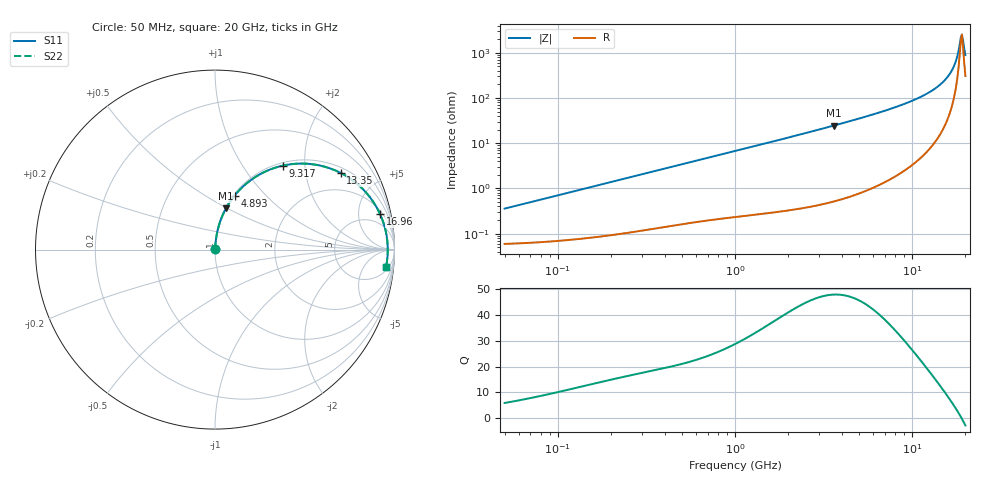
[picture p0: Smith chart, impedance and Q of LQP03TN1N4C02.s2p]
!Murata Part Number: LQP03TN1N4C02
!These Parameters are Measured in Series Mode Connection
!  o--[Z]--o
!Port1  Port2
!  o-------o
!Freq. Start=50[MHz] Stop=20[GHz], 401[Steps]
# Hz S RI R 50
!Freq.(Hz) S11(Real) S11(Imag) S21(Real) S21(Imag) S12(Real) S12(Imag) S22(Real) S22(Imag)
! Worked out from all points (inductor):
!   401 points, 50 MHz to 20 GHz, reference 50 ohm
!   read as one part in series: L = 1.12 nH near 51.52 MHz
!   highest Q = 47.7 at 3.626 GHz (marker M1), where L = 1.08 nH
!   self-resonance near 18.84 GHz
!   S11 on the Smith chart (normalised r, x): 50 MHz: 1.00, +0.01; 4.893 GHz: 1.01, +0.68; 9.317 GHz: 1.05, +1.55; 13.35 GHz: 1.20, +3.14; 16.96 GHz: 2.54, +8.71; 20 GHz: 7, -17
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5e7  0.000604 0.00352  0.9994 -0.00352  0.9994 -0.00352  0.000604 0.00352
1.364002e8  0.000862 0.00948  0.9991 -0.00948  0.9991 -0.00948  0.000862 0.00948
3.721004e8  0.00198 0.0253  0.998 -0.0253  0.998 -0.0253  0.00198 0.0253
1e9  0.00672 0.0661  0.9933 -0.0661  0.9933 -0.0661  0.00672 0.0661
2.728004e9  0.0359 0.1755  0.9641 -0.1755  0.9641 -0.1755  0.0359 0.1755
3.626126e9  0.0614 0.2298  0.9386 -0.2298  0.9386 -0.2298  0.0614 0.2298
4.89267e9  0.1093 0.3014  0.8907 -0.3014  0.8907 -0.3014  0.1093 0.3014
6.125241e9  0.1693 0.3632  0.8307 -0.3632  0.8307 -0.3632  0.1693 0.3632
7.442007e9  0.2471 0.4178  0.7529 -0.4178  0.7529 -0.4178  0.2471 0.4178
9.316812e9  0.3789 0.4681  0.6211 -0.4681  0.6211 -0.4681  0.3789 0.4681
1.131968e10  0.5378 0.4763  0.4622 -0.4763  0.4622 -0.4763  0.5378 0.4763
1.334722e10  0.7003 0.4272  0.2997 -0.4272  0.2997 -0.4272  0.7003 0.4272
1.527346e10  0.8349 0.3253  0.1651 -0.3253  0.1651 -0.3253  0.8349 0.3253
1.621653e10  0.8871 0.2576  0.1129 -0.2576  0.1129 -0.2576  0.8871 0.2576
1.696185e10  0.9199 0.197  0.0801 -0.197  0.0801 -0.197  0.9199 0.197
1.774144e10  0.945 0.1279  0.055 -0.1279  0.055 -0.1279  0.945 0.1279
1.800918e10  0.9512 0.103  0.0488 -0.103  0.0488 -0.103  0.9512 0.103
1.855685e10  0.9598 0.0504  0.0402 -0.0504  0.0402 -0.0504  0.9598 0.0504
1.88369e10  0.962 0.0227  0.038 -0.0227  0.038 -0.0227  0.962 0.0227
1.912117e10  0.9625 -0.00587  0.0375 0.00587  0.0375 0.00587  0.9625 -0.00587
1.940974e10  0.9613 -0.0353  0.0387 0.0353  0.0387 0.0353  0.9613 -0.0353
2e10  0.9529 -0.0968  0.0471 0.0968  0.0471 0.0968  0.9529 -0.0968
